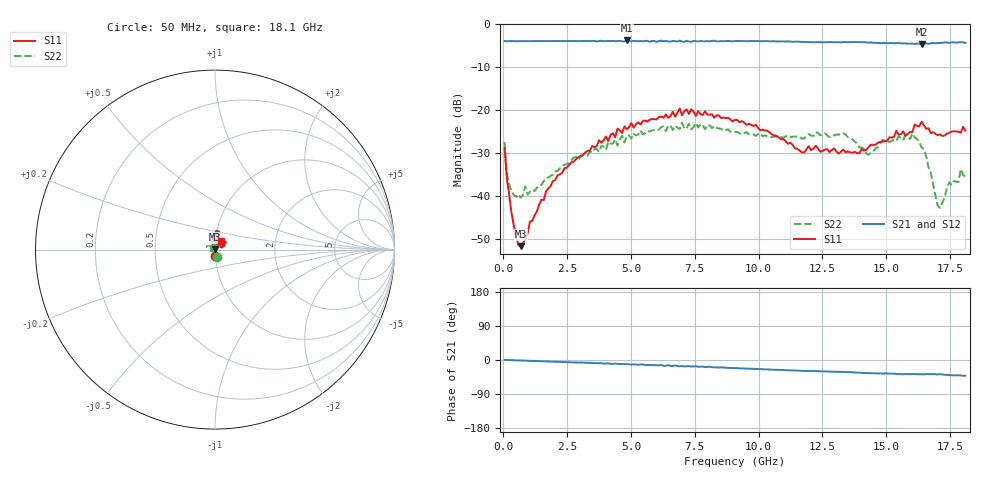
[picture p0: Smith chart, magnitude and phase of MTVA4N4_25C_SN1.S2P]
! Network Analyzer HP8720D.06.14 Serial No. US36140669
! 28 Jun 2005  10:02:40
! Frequency  S11  S21  S12  S22
# HZ  S  DB R 50
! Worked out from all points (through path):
!   201 points, 50 MHz to 18.1 GHz, reference 50 ohm
!   highest |S21| = -3.78 dB at 4.833 GHz (marker M1); lowest = -4.7 dB at 16.39 GHz (marker M2)
!   group delay of S21, straight-line fit = 6.54 ps
!   lowest |S11| = -51.6 dB at 681.8 MHz (marker M3), VSWR 1.01, Z = 49.7 + j0.0673 ohm
!   |S11| at or under -10 dB: start of sweep to end of sweep
!   |S22| runs from -42.7 to -22.9 dB; largest |S21 - S12| = 0.019
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5e7  -28.87 -86.5  -3.92 0.4  -3.94 0.5  -27.43 -77.9
1.4025e8  -35.99 -94.6  -3.98 -0.0  -3.97 -0.0  -34.91 -116.0
2.305e8  -39.73 -99.6  -3.95 -0.3  -3.94 -0.3  -37.28 -131.7
5.0125e8  -49.56 -138.9  -3.95 -1.1  -3.94 -1.0  -40.12 -169.2
6.8175e8  -51.63 165.1  -3.94 -1.3  -3.95 -1.4  -40.36 178.4
1.94525e9  -36.45 74.1  -3.93 -4.2  -3.93 -4.3  -35.00 122.5
3.1185e9  -30.42 73.6  -3.91 -6.8  -3.94 -7.1  -30.40 118.3
4.83325e9  -24.47 78.1  -3.78 -10.8  -3.86 -11.4  -26.05 95.1
6.09675e9  -21.60 77.0  -3.91 -14.1  -3.85 -14.1  -24.52 88.8
6.909e9  -19.59 83.6  -3.81 -16.8  -3.91 -16.1  -24.39 79.2
9.075e9  -22.20 94.9  -3.92 -21.2  -3.91 -21.4  -25.03 68.7
1.21435e10  -29.00 96.2  -4.20 -28.9  -4.17 -29.2  -26.01 79.5
1.331675e10  -29.12 64.2  -4.16 -31.5  -4.18 -31.7  -25.35 77.6
1.43095e10  -28.55 21.3  -4.28 -34.8  -4.24 -35.1  -30.36 90.5
1.512175e10  -26.31 24.1  -4.42 -36.1  -4.33 -36.0  -27.42 94.0
1.602425e10  -25.09 37.9  -4.49 -36.9  -4.60 -38.3  -25.42 63.9
1.638525e10  -22.67 32.9  -4.66 -37.6  -4.49 -37.6  -28.69 42.5
1.710725e10  -25.65 42.4  -4.37 -37.5  -4.33 -38.1  -42.74 88.8
1.746825e10  -25.29 51.7  -4.33 -39.5  -4.34 -39.4  -36.78 121.9
1.782925e10  -24.99 57.8  -4.23 -40.3  -4.25 -40.4  -36.77 143.5
1.79195e10  -25.24 58.5  -4.16 -41.1  -4.05 -40.8  -33.72 139.3
1.81e10  -24.80 57.4  -4.35 -41.5  -4.36 -42.5  -35.50 143.0
